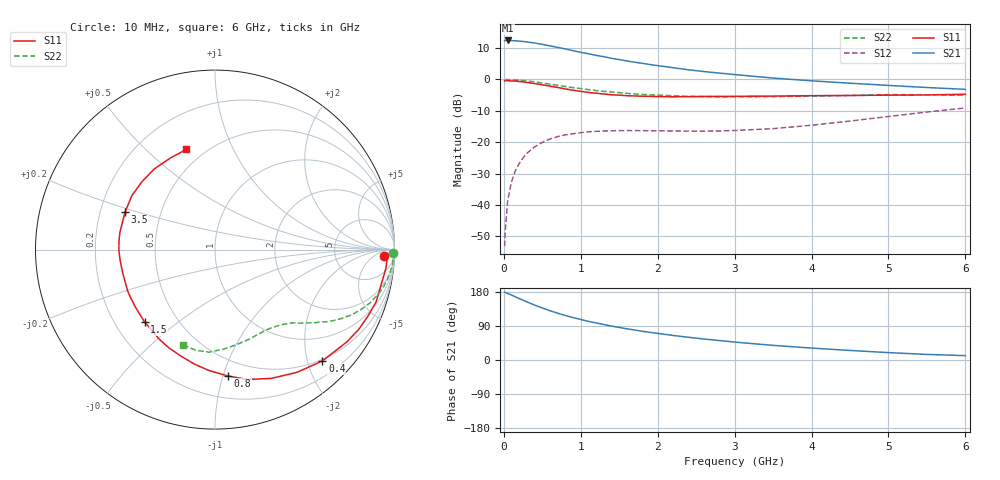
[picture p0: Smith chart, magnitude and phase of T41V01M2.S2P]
! Infineon Technologies  Discrete & RF Semiconductors
! BFR182T
! Si NPN RF Bipolar Junction Transistor in SC75
! VCE = 1 V  IC = 1.2 mA
! Common Emitter S-Parameters:  October  1999
# GHz  S  MA  R  50
!  f  S11  S21  S12  S22
! GHz  MAG  ANG  MAG  ANG  MAG  ANG  MAG  ANG
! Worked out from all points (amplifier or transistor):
!   36 points, 10 MHz to 6 GHz, reference 50 ohm
!   highest |S21| = 12.4 dB at 50 MHz (marker M1)
!   |S21| within 3 dB of that: start of sweep to 853.9 MHz
!   unconditionally stable (mu >= 1): 2.205 GHz to 4.843 GHz
!   at 250 MHz: K = 0.10, MSG = 18.6 dB, |S12| = -25.0 dB
!   at 1.4 GHz: K = 0.66, MSG = 11.6 dB, |S12| = -16.4 dB
!   at 6 GHz: K = 0.91, MSG = 3.0 dB, |S12| = -9.1 dB
!   S11 on the Smith chart (normalised r, x): 10 MHz: 23, -16; 400 MHz: 0.47, -2.27; 800 MHz: 0.37, -1.04; 1.5 GHz: 0.33, -0.38; 3.5 GHz: 0.31, +0.18; 6 GHz: 0.40, +0.67
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0.01  0.9445 -2.3  4.159 178.7  0.0022 73.0  0.9895 -1.2
0.02  0.9636 -1.2  4.18 178.5  0.0041 94.0  0.9978 -1.1
0.05  0.9582 -6.1  4.191 175.6  0.0117 90.5  0.9944 -2.5
0.1  0.9467 -11.5  4.156 171.4  0.0235 83.2  0.9922 -5.1
0.15  0.9437 -18.0  4.144 166.6  0.0351 79.3  0.983 -7.6
0.25  0.916 -29.0  4.039 157.8  0.0563 73.3  0.9622 -12.3
0.3  0.8971 -34.9  3.964 153.4  0.0667 70.1  0.9484 -14.5
0.4  0.8621 -46.0  3.815 144.9  0.0843 63.8  0.9154 -18.8
0.5  0.8225 -56.2  3.63 137.3  0.0997 58.4  0.8796 -22.3
0.6  0.7835 -66.3  3.435 130.0  0.1125 53.3  0.8435 -25.5
0.8  0.7077 -84.2  3.072 117.4  0.1309 45.5  0.7729 -30.7
0.9  0.6739 -93.0  2.88 111.9  0.1366 42.1  0.7418 -32.8
1.1  0.6216 -108.2  2.572 101.8  0.1466 37.0  0.6897 -36.2
1.3  0.5874 -122.1  2.308 93.5  0.151 33.3  0.647 -39.1
1.5  0.5628 -134.2  2.077 85.9  0.1528 31.0  0.6164 -41.6
1.8  0.541 -150.4  1.812 75.8  0.1532 28.9  0.578 -45.5
2.2  0.5303 -166.6  1.541 64.8  0.1511 29.6  0.5513 -50.2
2.8  0.5372 174.6  1.265 51.3  0.151 34.4  0.5294 -58.9
3.5  0.543 157.4  1.054 38.6  0.1646 43.5  0.5341 -69.2
4.5  0.5556 137.4  0.873 25.2  0.2174 52.8  0.5568 -85.2
5.5  0.5675 116.1  0.745 14.7  0.3028 53.2  0.5711 -100.9
6  0.5807 105.9  0.696 11.5  0.3519 50.6  0.5601 -108.4
